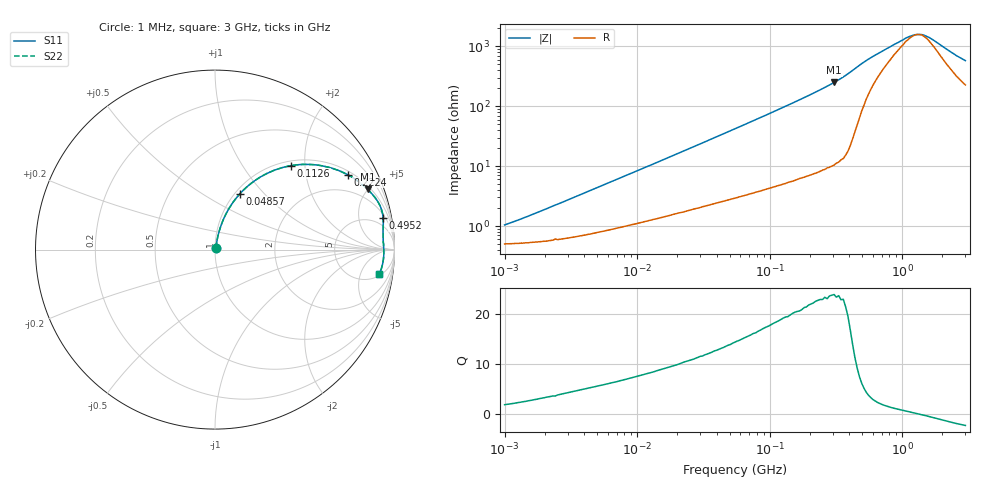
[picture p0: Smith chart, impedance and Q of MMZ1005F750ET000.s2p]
! S-parameter Generated by TDK Corporation
! Copyright(C) 2016 TDK Corporation.
! All Rights Reserved.
! TDK P/N: MMZ1005F750ET000 (Chip Beads)
! Property: |Z|=75¶ at 100MHz
! Size(LxWxT): 1x0.5x0.5mm, 0.039x0.02x0.02inches
! Model Type: s2p (Touchstone File Format Version 1.0)
! Frequency: DC=Yes Start=1MHz Stop=3000MHz 202points Log-sweep
! Note: This model was converted from impedance.
! Model Generated on May. 16, 2016
! Hash(MD5):
! Port Assignments:
!  1 ---@@@--- 2
! Applicable Conditions:
!  Temperature = 25 degC
!  DC Bias Current = 0 A
!  Small Signal Operation
! Terms and conditions regarding TDK Simulation Models
! (1)This simulation model is being provided solely for informational purposes. Please refer to the specifications of the products in terms of detailed characteristics of such products.
! (2)In no event shall TDK Corporation of any of its subsidiaries be liable for any loss or damage arising, directly or indirectly,
!  From any information contained in this simulation model, including, but not limited to loss or damages arising from any inaccuracies, omissions or errors in connection with such information.
! (3)Any and all copyrights on this simulation model are owned by TDK Corporation.
!  Duplication or redistribution of this simulation model without prior written permission from TDK Corporation is prohibited.
! (4)This simulation model is subject to any modification or change without any prior notice.
! (5)Neither TDK Corporation nor any of its subsidiaries shall make any warranty, express or implied,
!  Including but not limited to the correctness, implied warranties of merchantability and fitness for a particular purpose with respect to this simulation models.
! (6)The use of this simulation model shall be deemed to have consented to the terms and conditions hereof.
# MHz S MA R 50
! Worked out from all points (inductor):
!   201 points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, 1 MHz to 3 GHz, reference 50 ohm
!   read as one part in series: L = 143 nH near 1.823 MHz
!   highest Q = 23.7 at 306.3 MHz (marker M1), where L = 129 nH
!   self-resonance near 1.311 GHz
!   S11 on the Smith chart (normalised r, x): 1 MHz: 1.01, +0.02; 48.57 MHz: 1.05, +0.75; 112.6 MHz: 1.09, +1.70; 222.4 MHz: 1.15, +3.44; 495.2 MHz: 3, +10; 3 GHz: 6, -11
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1  0.01038 60.7  0.995 -0.5  0.995 -0.5  0.01038 60.7
3.900413  0.03454 76.5  0.9925 -1.9  0.9925 -1.9  0.03454 76.5
8.017732  0.06712 77.9  0.9881 -3.8  0.9881 -3.8  0.06712 77.9
14.61624  0.1168 76.8  0.98 -6.7  0.98 -6.7  0.1168 76.8
28.86629  0.2175 72.4  0.9571 -12.5  0.9571 -12.5  0.2175 72.4
48.57399  0.3425 65.9  0.915 -20.0  0.915 -20.0  0.3425 65.9
54.77226  0.3782 63.8  0.8998 -22.2  0.8998 -22.2  0.3782 63.8
78.52918  0.4992 56.6  0.8363 -29.9  0.8363 -29.9  0.4992 56.6
112.5904  0.6318 47.8  0.7416 -39.1  0.7416 -39.1  0.6318 47.8
155.0909  0.7444 39.2  0.6322 -48.0  0.6322 -48.0  0.7444 39.2
213.6344  0.8383 30.5  0.5087 -56.9  0.5087 -56.9  0.8383 30.5
222.3601  0.8485 29.5  0.493 -58.0  0.493 -58.0  0.8485 29.5
306.2963  0.9149 21.5  0.3673 -66.1  0.3673 -66.1  0.9149 21.5
374.1707  0.9439 16.8  0.2892 -70.5  0.2892 -70.5  0.9439 16.8
495.1867  0.9532 10.5  0.1852 -70.2  0.1852 -70.2  0.9532 10.5
800.5644  0.9394 4.5  0.09726 -49.3  0.09726 -49.3  0.9394 4.5
1147.801  0.9397 1.2  0.0638 -18.3  0.0638 -18.3  0.9397 1.2
1243.477  0.9402 0.5  0.06037 -7.8  0.06037 -7.8  0.9402 0.5
1402.151  0.9411 -0.6  0.05982 9.5  0.05982 9.5  0.9411 -0.6
1645.649  0.9408 -2.2  0.06964 30.8  0.06964 30.8  0.9408 -2.2
2556.106  0.9324 -6.8  0.1326 56.0  0.1326 56.0  0.9324 -6.8
3000  0.9258 -8.5  0.1607 58.4  0.1607 58.4  0.9258 -8.5
